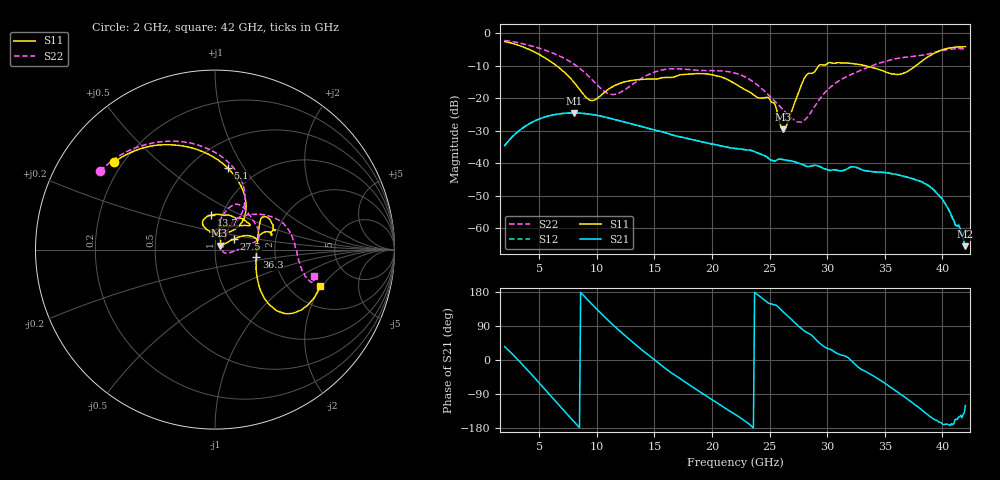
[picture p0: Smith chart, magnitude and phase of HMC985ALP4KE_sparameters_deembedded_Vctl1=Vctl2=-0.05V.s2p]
!s2p File: Measurements: S11, S21, S12, S22
# GHz S dB R 50.0
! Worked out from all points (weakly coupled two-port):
!   401 points, 2 GHz to 42 GHz, reference 50 ohm
!   highest |S21| = -24.54 dB at 8 GHz (marker M1); lowest = -65.6 dB at 42 GHz (marker M2)
!   lowest |S11| = -29.6 dB at 26.2 GHz (marker M3), VSWR 1.07, Z = 52.5 + j2.24 ohm
!   |S11| at or under -10 dB: 6.504 GHz to 29.28 GHz (22.77 GHz wide, 127 % of centre); 33.32 GHz to 37.71 GHz (4.389 GHz wide, 12.4 % of centre)
!   |S22| runs from -27.4 to -2.2 dB; largest |S21 - S12| = 0.00014
!   S11 on the Smith chart (normalised r, x): 2 GHz: 0.17, +0.36; 5.1 GHz: 0.74, +0.85; 13.7 GHz: 0.89, +0.35; 27.5 GHz: 1.23, +0.15; 36.3 GHz: 1.59, -0.14; 42 GHz: 2.90, -1.91
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2  -2.56 139.2  -34.62 35.4  -34.63 35.4  -2.22 145.6
3.5  -4.08 111.2  -29.37 -10.4  -29.37 -10.4  -3.16 122.0
5.1  -6.74 81.2  -26.27 -63.8  -26.28 -63.8  -4.71 97.6
8  -15.01 44.8  -24.54 -162.0  -24.55 -162.0  -9.45 60.2
8.7  -18.19 51.9  -24.64 175.1  -24.65 175.1  -11.33 54.8
9.7  -20.69 88.2  -25.07 143.4  -25.08 143.4  -14.68 52.2
11.2  -16.82 116.0  -26.24 98.6  -26.24 98.6  -18.79 66.9
13.7  -14.28 96.7  -28.56 32.1  -28.56 32.1  -14.29 77.2
15.4  -13.94 73.1  -30.13 -8.8  -30.13 -8.7  -11.52 68.4
19.4  -12.52 34.9  -33.65 -92.8  -33.66 -92.9  -11.48 34.2
22  -15.53 52.4  -35.47 -142.8  -35.49 -142.9  -12.26 13.2
25  -20.21 97.1  -38.86 148.6  -38.86 148.7  -19.36 -4.5
26.2  -29.60 40.1  -38.95 126.5  -38.94 126.4  -23.67 -17.4
27.5  -18.41 29.1  -39.99 89.7  -40.02 89.6  -27.30 -4.7
28.1  -13.38 20.5  -40.79 74.8  -40.81 74.6  -26.60 20.4
28.7  -12.31 12.6  -40.84 63.8  -40.77 63.5  -23.71 39.6
31  -9.09 23.2  -42.32 15.8  -42.28 16.1  -14.69 57.2
33.3  -9.98 34.3  -42.37 -29.8  -42.36 -29.9  -10.84 43.0
35.4  -12.29 12.4  -43.09 -70.0  -43.15 -70.0  -8.32 26.2
36.3  -12.60 -10.1  -43.75 -89.1  -43.73 -88.9  -7.64 18.2
39.5  -5.82 -43.3  -49.22 -158.7  -49.17 -159.2  -5.75 -15.1
42  -4.15 -19.0  -65.58 -120.2  -64.66 -116.9  -4.88 -15.0
